|   IBIS file stm32l496_4a6_ufbga169.ibs
[IBIS ver]   4.2
[File name]   stm32l496_4a6_ufbga169.ibs
[File Rev]   4.0
[Date]   08-10-2018
[Source]   Data Created at STMicroelectronics
[Notes]   File originated from ELDO simulations.
[Disclaimer]  This information is for modeling purpose only and is
   not guaranteed.
   The information is subject to change without notice.
[Copyright]   Copyright 2018 STMicroelectronics Inc.
|   Component stm32l496_4a6_ufbga169
[Component] stm32l496_4a6_ufbga169
[Manufacturer] STMicroelectronics
[Package]
| variable   typ   min   max
R_pkg   0.0   0.0   0.0
L_pkg   0.0H   0.0H   0.0H
C_pkg   0.0F   0.0F   0.0F
[Pin]  signal_name   model_name   R_pin   L_pin   C_pin
A10 PA14 io8prog2m25m50m120m_sudq_ft
A11 PA13 io8prog2m25m50m120m_sudq_ft
A12 PI0 io8prog2m25m50m120m_sudq_ft
A13 PH14 io8prog2m25m50m120m_sudq_ft
A2 PH2 io8prog2m25m50m120m_sudq_ft
A3 VDD POWER
A4 PE0 io8prog2m25m50m120m_sudq_ft
A5 PB4 io8prog2m25m50m120m_sudq_i2c_ft
A6 PB3 io8prog2m25m50m120m_sudq_ft
A7 VSS GND
A8 VDD POWER
A9 PA15 io8prog2m25m50m120m_sudq_ft
B1 PI9 io8prog2m25m50m120m_sudq_ft
B10 PI2 io8prog2m25m50m120m_sudq_ft
B11 PI1 io8prog2m25m50m120m_sudq_ft
B12 PH15 io8prog2m25m50m120m_sudq_ft
B13 PH12 io8prog2m25m50m120m_sudq_ft
B2 PI7 io8prog2m25m50m120m_sudq_ft
B3 VSS GND
B4 PE1 io8prog2m25m50m120m_sudq_ft
B5 PB5 io8prog2m25m50m120m_sudq_ft
B6 VDDIO2 POWER
B7 PG9 io8prog2m25m50m120m_sudq_ft
B8 PD0 io8prog2m25m50m120m_sudq_ft
B9 PI6 io8prog2m25m50m120m_sudq_ft
C1 VDD POWER
C10 PI3 io8prog2m25m50m120m_sudq_ft
C11 PI8 io8prog2m25m50m120m_sudq_ft
C12 VSS GND
C13 VDD POWER
C2 VSS GND
C3 PI11 io8prog2m25m50m120m_sudq_ft
C4 PB8 io8prog2m25m50m120m_sudq_i2c_ft
C5 PB6 io8prog2m25m50m120m_sudq_i2c_ft
C6 PG15 io8prog2m25m50m120m_sudq_ft
C7 PD4 io8prog2m25m50m120m_sudq_ft
C8 PD1 io8prog2m25m50m120m_sudq_ft
C9 PH13 io8prog2m25m50m120m_sudq_ft
D1 PE4 io8prog2m25m50m120m_sudq_ft
D10 PI4 io8prog2m25m50m120m_sudq_ft
D11 PH9 io8prog2m25m50m120m_sudq_ft
D12 PH7 io8prog2m25m50m120m_sudq_i2c_ft
D13 PA12 io8usblsfs_otg2
D2 PE3 io8prog2m25m50m120m_sudq_ft
D3 PE2 io8prog2m25m50m120m_sudq_ft
D4 PB9 io8prog2m25m50m120m_sudq_i2c_ft
D5 PB7 io8prog2m25m50m120m_sudq_i2c_ft
D6 PG10 io8prog2m25m50m120m_sudq_ft
D7 PD5 io8prog2m25m50m120m_sudq_ft
D8 PD2 io8prog2m25m50m120m_sudq_ft
D9 PC10 io8prog2m25m50m120m_sudq_ft
E1 PC13 io8prog2m25m50m120m_sudq_ft
E10 PI5 io8prog2m25m50m120m_sudq_ft
E11 PH6 io8prog2m25m50m120m_sudq_ft
E12 VDDUSB POWER
E13 PA11 io8usblsfs_otg2
E2 VBAT POWER
E3 PE6 io8prog2m25m50m120m_sudq_ft
E4 PE5 io8prog2m25m50m120m_sudq_ft
E5 PH3-BOOT0 io8prog2m25m50m120m_sudq_ft
E6 PG11 io8prog2m25m50m120m_sudq_ft
E7 PD6 io8prog2m25m50m120m_sudq_ft
E8 PD3 io8prog2m25m50m120m_sudq_ft
E9 PC11 io8prog2m25m50m120m_sudq_ft
F1 PC14-OSC32_IN io8prog2m25m50m120m_sudq_ft
F10 PA9 POWER
F11 PC6 io8prog2m25m50m120m_sudq_ft
F12 VDDIO2 POWER
F13 VSS GND
F2 VSS GND
F3 PF2 io8prog2m25m50m120m_sudq_ft
F4 PF1 io8prog2m25m50m120m_sudq_i2c_ft
F5 PF0 io8prog2m25m50m120m_sudq_i2c_ft
F6 PG12 io8prog2m25m50m120m_sudq_ft
F7 PD7 io8prog2m25m50m120m_sudq_ft
F8 PC12 io8prog2m25m50m120m_sudq_ft
F9 PA10 io8usb_id_otg20_lcd4_ft_ms
G1 PC15-OSC32_OUT io8prog2m25m50m120m_sudq_ft
G10 PC8 io8prog2m25m50m120m_sudq_ft
G11 PG6 io8prog2m25m50m120m_sudq_ft
G12 PC7 io8prog2m25m50m120m_sudq_ft
G13 VDD POWER
G2 VDD POWER
G3 PF3 io8prog2m25m50m120m_sudq_ft
G4 PF4 io8prog2m25m50m120m_sudq_ft
G5 PF5 io8prog2m25m50m120m_sudq_ft
G6 PG14 io8prog2m25m50m120m_sudq_i2c_ft
G7 PG13 io8prog2m25m50m120m_sudq_i2c_ft
G8 PA8 io8w_swp_lcd4_ft
G9 PC9 io8prog2m25m50m120m_sudq_i2c_ft
H1 PH0-OSC_IN io8prog2m25m50m120m_sudq_ft
H10 PG7 io8prog2m25m50m120m_sudq_i2c_ft
H11 PD15 io8prog2m25m50m120m_sudq_ft
H12 VSS GND
H13 VDD POWER
H2 VSS GND
H3 NRST ioreset_ft_v33
H4 PF10 io8prog2m25m50m120m_sudq_ft
H5 PC4 io8prog2m25m50m120m_sudq_ft
H6 PG1 io8prog2m25m50m120m_sudq_ft
H7 PE10 io8prog2m25m50m120m_sudq_ft
H8 PB11 io8prog2m25m50m120m_sudq_i2c_ft
H9 PG8 io8prog2m25m50m120m_sudq_i2c_ft
J1 PH1-OSC_OUT io8prog2m25m50m120m_sudq_ft
J10 PG4 io8prog2m25m50m120m_sudq_ft
J11 PG3 io8prog2m25m50m120m_sudq_ft
J12 PG2 io8prog2m25m50m120m_sudq_ft
J13 PD10 io8prog2m25m50m120m_sudq_ft
J2 PC0 io8prog2m25m50m120m_sudq_i2c_ft
J3 PC1 io8prog2m25m50m120m_sudq_i2c_ft
J4 PC2 io8prog2m25m50m120m_sudq_ft
J5 PC5 io8prog2m25m50m120m_sudq_ft
J6 PG0 io8prog2m25m50m120m_sudq_ft
J7 PE9 io8prog2m25m50m120m_sudq_ft
J8 PE15 io8prog2m25m50m120m_sudq_ft
J9 PG5 io8prog2m25m50m120m_sudq_ft
K1 PC3 io8prog2m25m50m120m_sudq_ft
K10 PD14 io8prog2m25m50m120m_sudq_ft
K11 PD12 io8prog2m25m50m120m_sudq_i2c_ft
K12 PD11 io8prog2m25m50m120m_sudq_ft
K13 PD13 io8prog2m25m50m120m_sudq_i2c_ft
K2 VSSA_VREF- GND
K3 PA0 io8prog2m25m50m120m_sudq_ft
K4 PA5 io8prog2m25m50m120m_sudq_ft
K5 PB0 io8prog2m25m50m120m_sudq_ft
K6 PF15 io8prog2m25m50m120m_sudq_i2c_ft
K7 PE8 io8prog2m25m50m120m_sudq_ft
K8 PE14 io8prog2m25m50m120m_sudq_ft
K9 PH4 io8prog2m25m50m120m_sudq_i2c_ft
L1 VREF+ POWER
L10 PD9 io8prog2m25m50m120m_sudq_ft
L11 PD8 io8prog2m25m50m120m_sudq_ft
L12 VDD POWER
L13 VSS GND
L2 VDDA POWER
L3 PA4 io8prog2m25m50m120m_sudq_ft
L4 PA7 io8prog2m25m50m120m_sudq_i2c_ft
L5 PB1 io8prog2m25m50m120m_sudq_ft
L6 PF14 io8prog2m25m50m120m_sudq_i2c_ft
L7 PE7 io8prog2m25m50m120m_sudq_ft
L8 PE13 io8prog2m25m50m120m_sudq_ft
L9 PH5 io8prog2m25m50m120m_sudq_i2c_ft
M10 PH11 io8prog2m25m50m120m_sudq_ft
M11 VSS GND
M12 PB15 io8prog2m25m50m120m_sudq_ft
M13 PB14 io8prog2m25m50m120m_sudq_i2c_ft
M2 PA3 io8prog2m25m50m120m_sudq_ft
M3 VSS GND
M4 PA6 io8prog2m25m50m120m_sudq_ft
M5 PF11 io8prog2m25m50m120m_sudq_ft
M6 PF13 io8prog2m25m50m120m_sudq_ft
M7 VSS GND
M8 PE12 io8prog2m25m50m120m_sudq_ft
M9 PH10 io8prog2m25m50m120m_sudq_ft
N1 PA2 io8prog2m25m50m120m_sudq_ft
N10 PH8 io8prog2m25m50m120m_sudq_i2c_ft
N11 VDD POWER
N12 PB12 io8w_swp_lcd4_ft
N13 PB13 io8prog2m25m50m120m_sudq_i2c_ft
N2 PA1 io8prog2m25m50m120m_sudq_ft
N3 VDD POWER
N5 PB2 io8prog2m25m50m120m_sudq_ft
N6 PF12 io8prog2m25m50m120m_sudq_ft
N7 VDD io8prog2m25m50m120m_sudq_ft
N8 PE11 io8prog2m25m50m120m_sudq_ft
N9 PB10 io8prog2m25m50m120m_sudq_i2c_ft
[Diff Pin]   inv_pin   vdiff   tdelay_typ  tdelay_min  tdelay_max
D13 E13 200mV   NA   NA   NA
[Model Selector] io8usblsfs_otg2
usb_ls_pd  "USB Low Speed mode - Pull Down"
usb_ls_pu2  "USB Low Speed mode - Pull up 2"
usb_ls_pu  "USB Low Speed mode - Pull up"
usb_fs  "USB Low Speed mode"
usb_fs_pd  "USB Full Speed mode - Pull Down"
usb_fs_pu2  "USB Full Speed mode - Pull up 2"
usb_fs_pu  "USB Full Speed mode - Pull up"
[Model Selector] io8usb_id_otg20_lcd4_ft_ms
io8usbid_1v8_id_pu  "ID 1V8 range with pull up"
io8usbid_3v3_id_pu  "ID 3V3 range with pull up"
io8usbid_1v8_id  "ID 1V8 range"
io8usbid_3v3_id  "ID 3V3 range"
io8lsusbid_1v8_pd  "GPIO 1.8V range with pd io low speed"
io8lsusbid_1v8_pu  "GPIO 1.8V range with pu io low speed"
io8lsusbid_1v8  "GPIO 1.8V range io low speed"
io8lsusbid_3v3_pd  "GPIO 3.3V range with pd io low speed"
io8lsusbid_3v3_pu  "GPIO 3.3V range with pu io low speed"
io8lsusbid_3v3  "GPIO 3.3V range io low speed"
io8fsusbid_1v8_pd  "GPIO 1.8V range with pd io full speed"
io8fsusbid_1v8_pu  "GPIO 1.8V range with pu io full speed"
io8fsusbid_1v8  "GPIO 1.8V range io full speed"
io8fsusbid_3v3_pd  "GPIO 3.3V range with pd io full speed"
io8fsusbid_3v3_pu  "GPIO 3.3V range with pu io full speed"
io8fsusbid_3v3  "GPIO 3.3V range io full speed"
io8msusbid_1v8_pd  "GPIO 1.8V range with pd io medium speed"
io8msusbid_1v8_pu  "GPIO 1.8V range with pu io medium speed"
io8msusbid_1v8  "GPIO 1.8V range io medium speed"
io8msusbid_3v3_pd  "GPIO 3.3V range with pd io medium speed"
io8msusbid_3v3_pu  "GPIO 3.3V range with pu io medium speed"
io8msusbid_3v3  "GPIO 3.3V range io medium speed"
io8hsusbid_1v8_pd  "GPIO 1.8V range with pd io high speed"
io8hsusbid_1v8_pu  "GPIO 1.8V range with pu io high speed"
io8hsusbid_1v8  "GPIO 1.8V range io high speed"
io8hsusbid_3v3_pd  "GPIO 3.3V range with pd io high speed"
io8hsusbid_3v3_pu  "GPIO 3.3V range with pu io high speed"
io8hsusbid_3v3  "GPIO 3.3V range io high speed"
[Model Selector] io8w_swp_lcd4_ft
io8w_swp_classc  "Class C swp functionality"
io8w_swp_classb  "Class B swp functionality"
io8lsw_1v8_pd  "GPIO 1.8V range with pd io low speed"
io8lsw_1v8_pu  "GPIO 1.8V range with pu io low speed"
io8lsw_1v8  "GPIO 1.8V range io low speed"
io8lsw_3v3_pd  "GPIO 3.3V range with pd io low speed"
io8lsw_3v3_pu  "GPIO 3.3V range with pu io low speed"
io8lsw_3v3  "GPIO 3.3V range io low speed"
io8fsw_1v8_pd  "GPIO 1.8V range with pd io full speed"
io8fsw_1v8_pu  "GPIO 1.8V range with pu io full speed"
io8fsw_1v8  "GPIO 1.8V range io full speed"
io8fsw_3v3_pd  "GPIO 3.3V range with pd io full speed"
io8fsw_3v3_pu  "GPIO 3.3V range with pu io full speed"
io8fsw_3v3  "GPIO 3.3V range io full speed"
io8msw_1v8_pd  "GPIO 1.8V range with pd io medium speed"
io8msw_1v8_pu  "GPIO 1.8V range with pu io medium speed"
io8msw_1v8  "GPIO 1.8V range io medium speed"
io8msw_3v3_pd  "GPIO 3.3V range with pd io medium speed"
io8msw_3v3_pu  "GPIO 3.3V range with pu io medium speed"
io8msw_3v3  "GPIO 3.3V range io medium speed"
io8hsw_1v8_pd  "GPIO 1.8V range with pd io high speed"
io8hsw_1v8_pu  "GPIO 1.8V range with pu io high speed"
io8hsw_1v8  "GPIO 1.8V range io high speed"
io8hsw_3v3_pd  "GPIO 3.3V range with pd io high speed"
io8hsw_3v3_pu  "GPIO 3.3V range with pu io high speed"
io8hsw_3v3  "GPIO 3.3V range io high speed"
[Model Selector] io8prog2m25m50m120m_sudq_ft
iols8p_sudq_ft_pd_lv  "IO low speed, PD=40kOhm - 1P8V"
iols8p_sudq_ft_pu_lv  "IO low speed, PU=40kOhm - 1P8V"
iols8p_sudq_ft_lv  "IO low speed - 1P8V"
iols8p_sudq_ft_pd  "IO low speed, PD=40kOhm - 3P3V"
iols8p_sudq_ft_pu  "IO low speed, PU=40kOhm - 3P3V"
iols8p_sudq_ft  "IO low speed - 3P3V"
iofs8p_sudq_ft_pd_lv  "IO full speed, PD=40kOhm - 1P8V"
iofs8p_sudq_ft_pu_lv  "IO full speed, PU=40kOhm - 1P8V"
iofs8p_sudq_ft_lv  "IO full speed - 1P8V"
iofs8p_sudq_ft_pd  "IO full speed, PD=40kOhm - 3P3V"
iofs8p_sudq_ft_pu  "IO full speed, PU=40kOhm - 3P3V"
iofs8p_sudq_ft  "IO full speed - 3P3V"
ioms8p_sudq_ft_pd_lv  "IO medium speed, PD=40kOhm - 1P8V"
ioms8p_sudq_ft_pu_lv  "IO medium speed, PU=40kOhm - 1P8V"
ioms8p_sudq_ft_lv  "IO medium speed - 1P8V"
ioms8p_sudq_ft_pd  "IO medium speed, PD=40kOhm - 3P3V"
ioms8p_sudq_ft_pu  "IO medium speed, PU=40kOhm - 3P3V"
ioms8p_sudq_ft  "IO medium speed - 3P3V"
iohs8p_sudq_ft_pd_lv  "IO high speed, PD=40kOhm - 1P8V"
iohs8p_sudq_ft_pu_lv  "IO high speed, PU=40kOhm - 1P8V"
iohs8p_sudq_ft_lv  "IO high speed - 1P8V"
iohs8p_sudq_ft_pd  "IO high speed, PD=40kOhm - 3P3V"
iohs8p_sudq_ft_pu  "IO high speed, PU=40kOhm - 3P3V"
iohs8p_sudq_ft  "IO high speed - 3P3V"
[Model Selector] io8prog2m25m50m120m_sudq_i2c_ft
io8prog_1v8_i2c_pd  "5V Tol GPIO 1.8V range i2c functionality with pull down"
io8prog_1v8_i2c_pu  "5V Tol GPIO 1.8V range i2c functionality with pull up"
io8prog_1v8_i2c  "5V Tol GPIO 1.8V range i2c functionality"
io8prog_3v3_i2c_pd  "5V Tol GPIO 3.3V range i2c functionality with pull down"
io8prog_3v3_i2c_pu  "5V Tol GPIO 3.3V range i2c functionality with pull up"
io8prog_3v3_i2c  "5V Tol GPIO 3.3V range i2c functionality"
io8ls_1v8_pd  "5V Tol GPIO 1.8V range with pd io low speed"
io8ls_1v8_pu  "5V Tol GPIO 1.8V range with pu io low speed"
io8ls_1v8  "5V Tol GPIO 1.8V range io low speed"
io8ls_3v3_pd  "5V Tol GPIO 3.3V range with pd io low speed"
io8ls_3v3_pu  "5V Tol GPIO 3.3V range with pu io low speed"
io8ls_3v3  "5V Tol GPIO 3.3V range io low speed"
io8fs_1v8_pd  "5V Tol GPIO 1.8V range with pd io full speed"
io8fs_1v8_pu  "5V Tol GPIO 1.8V range with pu io full speed"
io8fs_1v8  "5V Tol GPIO 1.8V range io full speed"
io8fs_3v3_pd  "5V Tol GPIO 3.3V range with pd io full speed"
io8fs_3v3_pu  "5V Tol GPIO 3.3V range with pu io full speed"
io8fs_3v3  "5V Tol GPIO 3.3V range io full speed"
io8ms_1v8_pd  "5V Tol GPIO 1.8V range with pd io medium speed"
io8ms_1v8_pu  "5V Tol GPIO 1.8V range with pu io medium speed"
io8ms_1v8  "5V Tol GPIO 1.8V range io medium speed"
io8ms_3v3_pd  "5V Tol GPIO 3.3V range with pd io medium speed"
io8ms_3v3_pu  "5V Tol GPIO 3.3V range with pu io medium speed"
io8ms_3v3  "5V Tol GPIO 3.3V range io medium speed"
io8hs_1v8_pd  "5V Tol GPIO 1.8V range with pd io high speed"
io8hs_1v8_pu  "5V Tol GPIO 1.8V range with pu io high speed"
io8hs_1v8  "5V Tol GPIO 1.8V range io high speed"
io8hs_3v3_pd  "5V Tol GPIO 3.3V range with pd io high speed"
io8hs_3v3_pu  "5V Tol GPIO 3.3V range with pu io high speed"
io8hs_3v3  "5V Tol GPIO 3.3V range io high speed"
[Model Selector] ioreset_ft_v33
ioreset_1v2_pu  "RESET 1.2V range with PU"
ioreset_1v2  "RESET 1.2V range"
ioreset_1v8_pu  "RESET 1.8V range with PU"
ioreset_1v8  "RESET 1.8V range"
ioreset_3v3_pu  "RESET 3.3V range with PU"
ioreset_3v3  "RESET 3.3V range"
| Models and submodels in the file (121): usb_ls_pd (I/O), usb_ls_pu2 (I/O), usb_ls_pu (I/O), usb_fs (I/O), usb_fs_pd (I/O), usb_fs_pu2 (I/O), usb_fs_pu (I/O), io8usbid_1v8_id_pu (Input), io8usbid_3v3_id_pu (Input), io8usbid_1v8_id (Input), io8usbid_3v3_id (Input), io8lsusbid_1v8_pd (I/O), io8lsusbid_1v8_pu (I/O), io8lsusbid_1v8 (I/O), io8lsusbid_3v3_pd (I/O), io8lsusbid_3v3_pu (I/O), io8lsusbid_3v3 (I/O), io8fsusbid_1v8_pd (I/O), io8fsusbid_1v8_pu (I/O), io8fsusbid_1v8 (I/O), io8fsusbid_3v3_pd (I/O), io8fsusbid_3v3_pu (I/O), io8fsusbid_3v3 (I/O), io8msusbid_1v8_pd (I/O), io8msusbid_1v8_pu (I/O), io8msusbid_1v8 (I/O), io8msusbid_3v3_pd (I/O), io8msusbid_3v3_pu (I/O), io8msusbid_3v3 (I/O), io8hsusbid_1v8_pd (I/O), io8hsusbid_1v8_pu (I/O), io8hsusbid_1v8 (I/O), io8hsusbid_3v3_pd (I/O), io8hsusbid_3v3_pu (I/O), io8hsusbid_3v3 (I/O), io8w_swp_classc (I/O), io8w_swp_classb (I/O), io8lsw_1v8_pd (I/O), io8lsw_1v8_pu (I/O), io8lsw_1v8 (I/O), io8lsw_3v3_pd (I/O), io8lsw_3v3_pu (I/O), io8lsw_3v3 (I/O), io8fsw_1v8_pd (I/O), io8fsw_1v8_pu (I/O), io8fsw_1v8 (I/O), io8fsw_3v3_pd (I/O), io8fsw_3v3_pu (I/O), io8fsw_3v3 (I/O), io8msw_1v8_pd (I/O), io8msw_1v8_pu (I/O), io8msw_1v8 (I/O), io8msw_3v3_pd (I/O), io8msw_3v3_pu (I/O), io8msw_3v3 (I/O), io8hsw_1v8_pd (I/O), io8hsw_1v8_pu (I/O), io8hsw_1v8 (I/O), io8hsw_3v3_pd (I/O), io8hsw_3v3_pu (I/O), io8hsw_3v3 (I/O), iols8p_sudq_ft_pd_lv (I/O), iols8p_sudq_ft_pu_lv (I/O), iols8p_sudq_ft_lv (I/O), iols8p_sudq_ft_pd (I/O), iols8p_sudq_ft_pu (I/O), iols8p_sudq_ft (I/O), iofs8p_sudq_ft_pd_lv (I/O), iofs8p_sudq_ft_pu_lv (I/O), iofs8p_sudq_ft_lv (I/O), iofs8p_sudq_ft_pd (I/O), iofs8p_sudq_ft_pu (I/O), iofs8p_sudq_ft (I/O), ioms8p_sudq_ft_pd_lv (I/O), ioms8p_sudq_ft_pu_lv (I/O), ioms8p_sudq_ft_lv (I/O), ioms8p_sudq_ft_pd (I/O), ioms8p_sudq_ft_pu (I/O), ioms8p_sudq_ft (I/O), iohs8p_sudq_ft_pd_lv (I/O)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
